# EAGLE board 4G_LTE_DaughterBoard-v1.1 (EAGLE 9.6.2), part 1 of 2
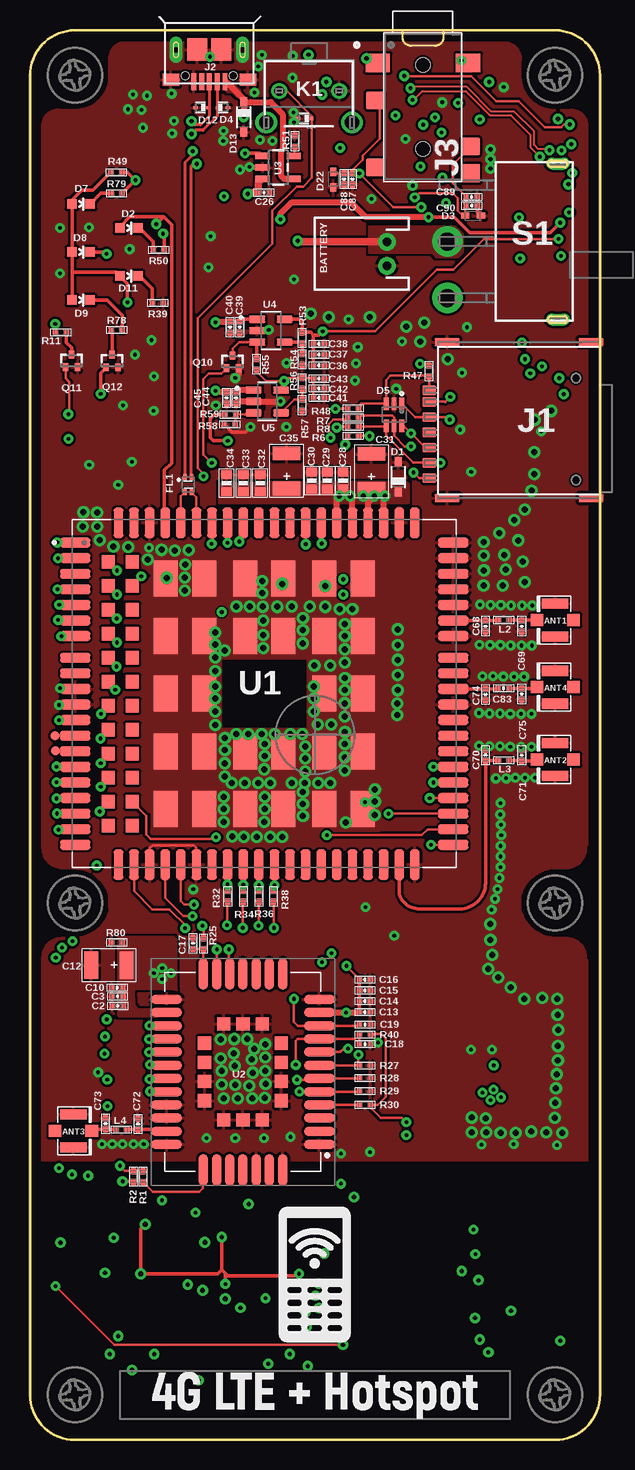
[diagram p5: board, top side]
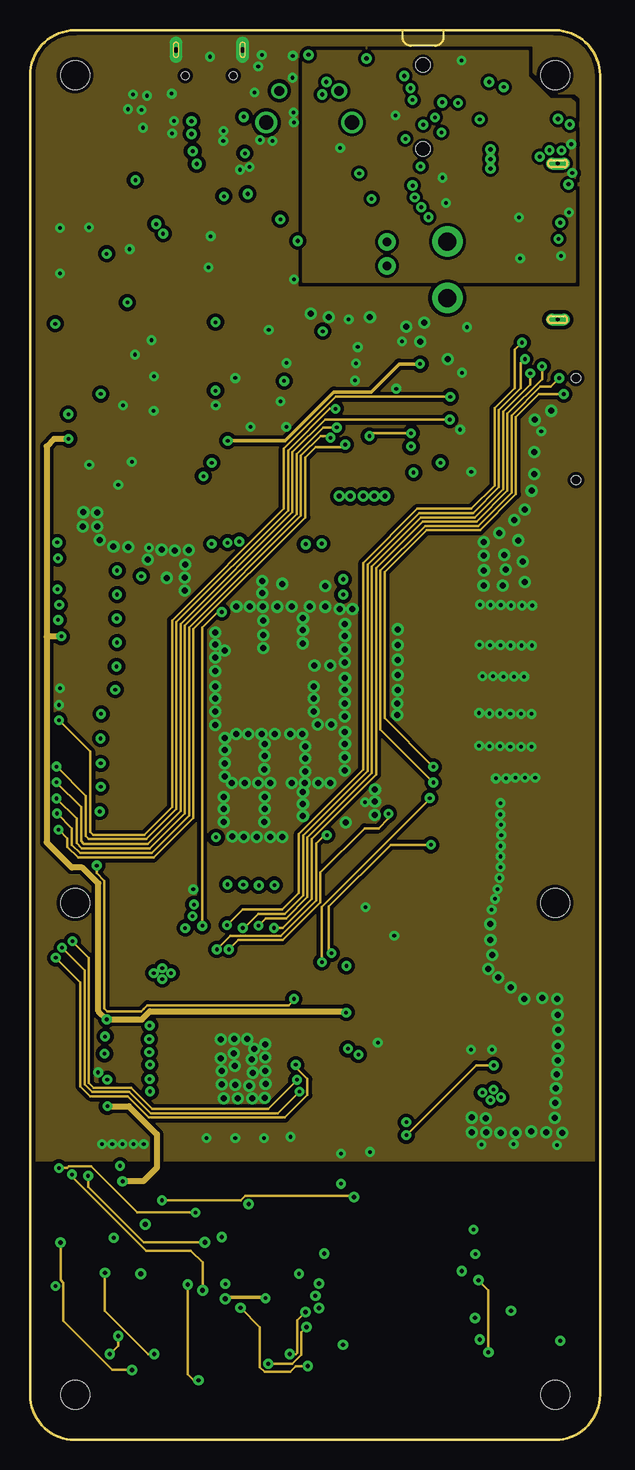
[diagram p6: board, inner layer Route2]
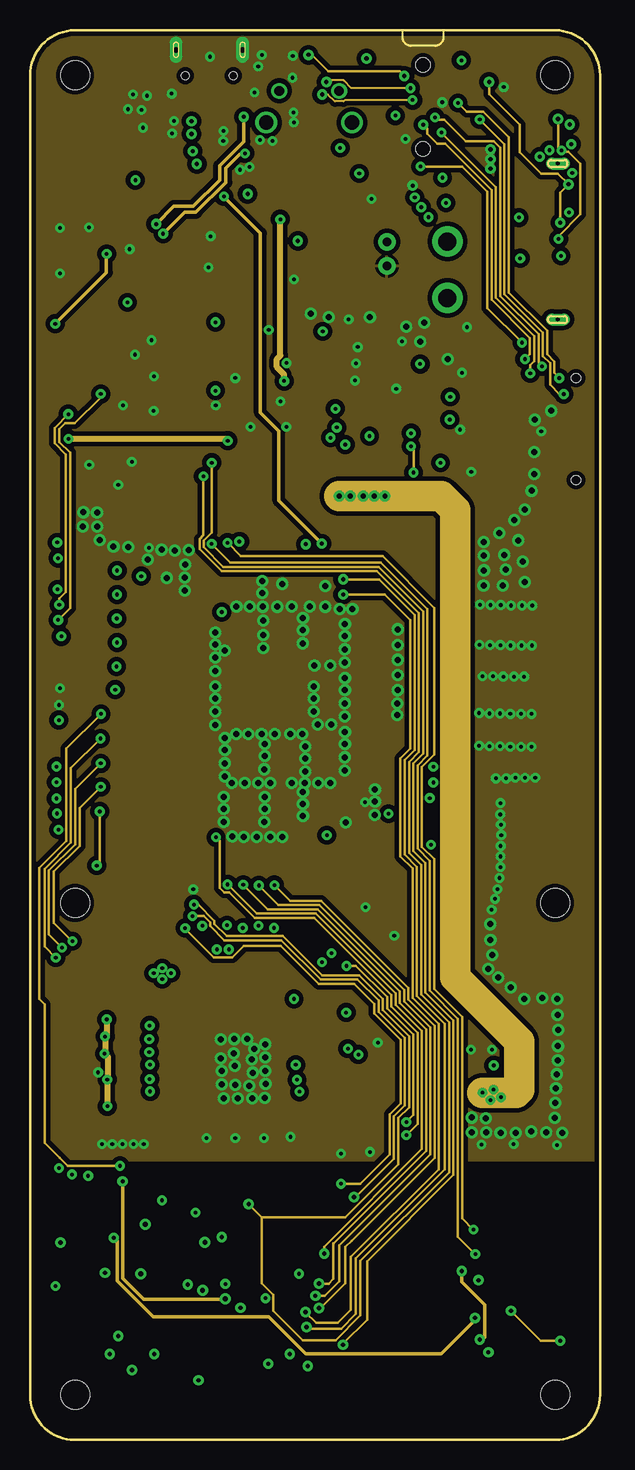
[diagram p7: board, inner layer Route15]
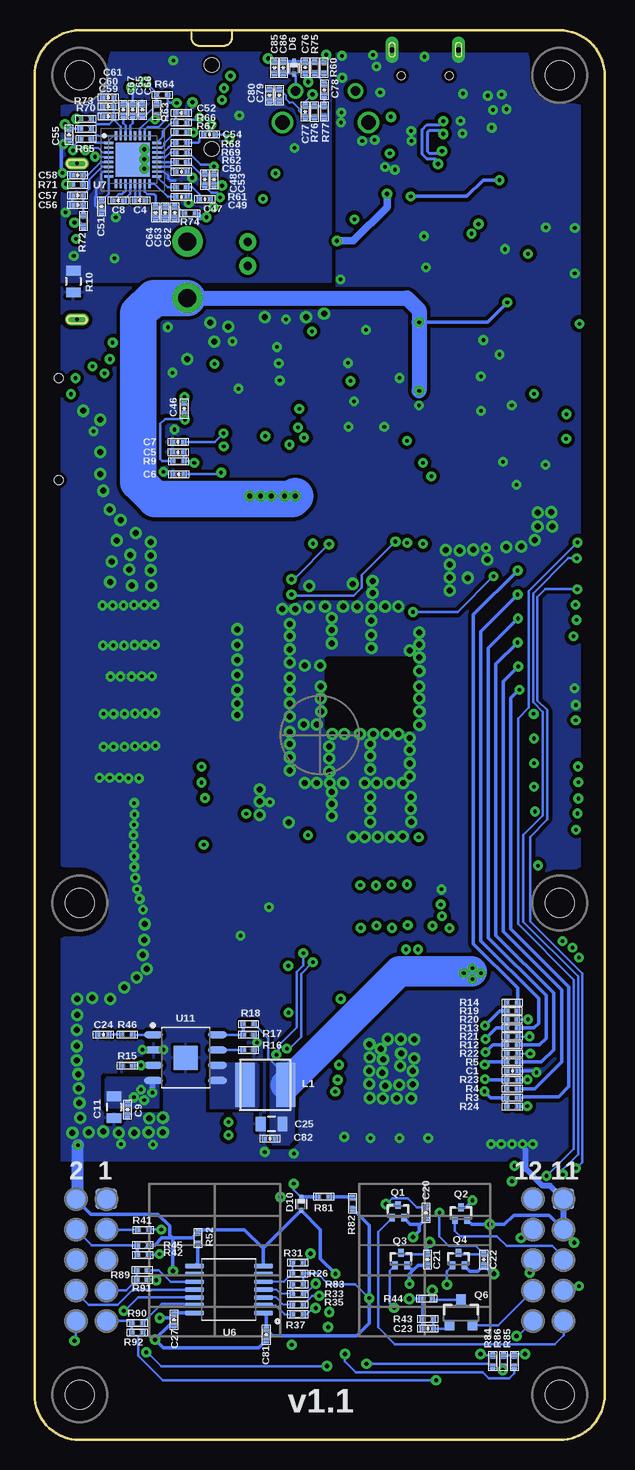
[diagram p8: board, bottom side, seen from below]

Size 47.5 x 117.5 mm. Coordinates in mm from the lower left corner, seen from the top.
Copper layers (1*2+15*16): Top 0.035mm / dielectric 1.5mm / Route2 0.035mm / dielectric 0.15mm / Route15 0.035mm / dielectric 0.2mm / Bottom 0.035mm
Design rules "4LDaughterBoards": minimum track width 6mil, minimum drill 0.3mm, track to track 6mil, track to pad 6mil, pad to pad 6mil, via to via 6mil, smd to smd 0mil, copper to edge 0.2mm, drill to drill 8mil, minimum pad ring 10mil, minimum via ring 10mil, stop-mask expansion 4mil, vias tented up to drill 25mil, thermal gap 10mil
Net classes: 1 USB_Data: width 0.261 mm, drill 0.305 mm, clearance 0.203 mm; 2 SDIO3.0: width 0.235 mm, drill 0.305 mm, clearance 0.305 mm
tRestrict: area 39.3,56.4 to 39.7,56.9; area 17.8,86.9 to 19.4,87.1; area 17.8,86 to 19.4,86.2
Milling: 5 lines

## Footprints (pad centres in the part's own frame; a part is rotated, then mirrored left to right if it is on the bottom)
U.FL = smd 2.2 x 0.85: 1 0,1.375; 2 0,-1.375 | smd 1.05 x 1: FEED 1.525,0; NC -1.525,0
JST-2-PTH = drill 0.7 pad 1.448: 1 -1,0; 2 1,0
0402-CAP = smd 0.508 x 0.508: 1 -0.457,0; 2 0.457,0
0805_CAP = smd 0.8 x 1.2: 1 -0.9,0; 2 0.9,0
AVX-B = smd 1.143 x 2.286: + -1.46,0; - 1.46,0
0603-CAP-L = smd 0.75 x 0.9: 1 -0.7,0; 2 0.7,0
SOD323 = smd 0.8 x 0.6: A 1.25,0; C -1.25,0
0603-LED = smd 0.8 x 0.8: A 0,-0.75; C 0,0.75
SOD523 = smd 0.7 x 0.5: A 0.7,0; C -0.6,0
SOD923 = smd 0.36 x 0.25: A 0.42,0; C -0.42,0
DIO_ESDA6V1-5W6 = smd 1.05 x 0.4: 1 -0.925,0.65; 2 -0.925,0; 3 -0.925,-0.65; 4 0.925,-0.65; 5 0.925,0; 6 0.925,0.65
SODFL1060X40N = smd 0.41 x 0.31: 1 -0.55,0; 2 0.55,0
SMD,1.25X1.0X0.5MM = smd 0.3 x 0.5: 1 -0.275,0.625; 2 0.275,0.625; 3 0.275,-0.625; 4 -0.275,-0.625
XUNPU-SMN-303_C266888 = smd 0.8 x 1.14: C1 0.256,7.48; C2 -2.285,7.48; C3 -4.825,7.48; C5 1.526,7.48; C6 -1.015,7.48; C7 -3.555,7.48; CD 2.476,7.48 | smd 0.7 x 2.1: P$1 -6.495,6; P$2 6.505,6; P$3 6.505,-6; P$4 -6.495,-6 | hole 0.75: -4.995,-4.75; 3.505,-4.75
B-SMD-5P-0.65SLOT = smd 0.406 x 1.4: 1 1.3,0; 2 0.65,0; 3 0,0; 4 -0.65,0; 5 -1.3,0 | smd 1.372 x 1.016: 6 -3.2,0.15; 7 3.2,0.15 | drill 0.45 pad 1.1 long: 8 2.775,2.65; 9 -2.775,2.65 | smd 1.651 x 1.9: 10 -1,2.667; 11 1,2.667 | hole 0.65: -2,0.5; 2,0.5
PJ-342-SMT_3.5MM = smd 1.524 x 2.032: 1 -3.678,-3.768; 2 -3.678,3.759 | smd 1.524 x 1.524: 3 -0.538,-3.988; 4 3.301,3.988; 5 5.037,-3.988; 6 5.52,3.988 | hole 1.2: -3.5,0; 3.51,0
3X6X5-90_DEGREE = drill 0.8: 1 -2.534,-0.964; 2 2.46,-0.964 | drill 1.2: ANCHOR1 -3.609,1.68; ANCHOR2 3.541,1.68
IND4018 = smd 1.6 x 3.7: 1 -1.7,0; 2 1.7,0
0402-IND = smd 0.508 x 0.508: 1 -0.457,0; 2 0.457,0
SC89 = smd 0.45 x 0.65: 1 -0.5,-0.525; 2 0.5,-0.525; 3 0,0.525
SOT23-3-L = smd 0.8 x 0.9: 1 -0.95,-1; 2 0.95,-1; 3 0,1.1
0402-RES = smd 0.508 x 0.508: 1 -0.457,0; 2 0.457,0
0805_RES = smd 0.8 x 1.2: 1 -0.9,0; 2 0.9,0
SWITCH_SPDT_PTH_90D_13X9.2MM = drill 1.5 pad 2.54: 2 -7.25,0; 3 -7.25,-4.7 | drill 0.3 pad 1 long: P$1 1.95,-6.5; P$2 1.95,6.5
PAD.03X.03 = smd 0.762 x 0.762: P$1 0,0
EC25EFA = smd 2.5 x 0.8: 1 -15.75,12.6; 2 -15.75,11.3; 3 -15.75,10; 4 -15.75,8.7; 5 -15.75,7.4; 6 -15.75,6.1; 7 -15.75,4.8; 8 -15.75,0.4; 9 -15.75,-0.9; 10 -15.75,-2.2; 11 -15.75,-3.5; 12 -15.75,-4.8; 13 -15.75,-6.1; 14 -15.75,-7.4; 15 -15.75,-8.7; 16 -15.75,-10; 17 -15.75,-11.3; 18 -15.75,-12.6; 37 15.75,-12.6; 38 15.75,-11.3; 39 15.75,-10; 40 15.75,-8.7; 41 15.75,-7.4; 42 15.75,-6.1; 43 15.75,-4.8; 44 15.75,-3.5; 45 15.75,-2.2; 46 15.75,-0.9; 47 15.75,0.4; 48 15.75,4.8; 49 15.75,6.1; 50 15.75,7.4; 51 15.75,8.7; 52 15.75,10; 53 15.75,11.3; 54 15.75,12.6; 141 -15.75,3; 142 -15.75,1.7; 143 15.75,1.7; 144 15.75,3 | smd 0.8 x 2.5: 19 -9.55,-14.25; 20 -8.25,-14.25; 21 -6.95,-14.25; 22 -5.65,-14.25; 23 -4.35,-14.25; 24 -3.05,-14.25; 25 -1.75,-14.25; 26 -0.45,-14.25; 27 0.85,-14.25; 28 2.15,-14.25; 29 3.45,-14.25; 30 4.75,-14.25; 31 6.05,-14.25; 32 7.35,-14.25; 33 8.65,-14.25; 34 9.95,-14.25; 35 11.25,-14.25; 36 12.55,-14.25; 55 12.55,14.25; 56 11.25,14.25; 57 9.95,14.25; 58 8.65,14.25; 59 7.35,14.25; 60 6.05,14.25; 61 4.75,14.25; 62 3.45,14.25; 63 2.15,14.25; 64 0.85,14.25; 65 -0.45,14.25; 66 -1.75,14.25; 67 -3.05,14.25; 68 -4.35,14.25; 69 -5.65,14.25; 70 -6.95,14.25; 71 -8.25,14.25; 72 -9.55,14.25; 113 -10.85,14.25; 114 -12.15,14.25; 115 -10.85,-14.25; 116 -12.15,-14.25 | smd 2 x 3: 85 8.2,9.6; 86 8.2,4.8; 87 8.2,0; 88 8.2,-4.8; 89 8.2,-9.6; 90 5,9.6; 91 5,4.8; 92 5,0; 93 5,-4.8; 94 5,-9.6; 95 1.6,9.6; 96 1.6,4.8; 97 1.6,-4.8; 98 1.6,-9.6; 99 -1.6,9.6; 100 -1.6,4.8; 101 -1.6,-4.8; 102 -1.6,-9.6; 103 -5,9.6; 104 -5,4.8; 105 -5,0; 106 -5,-4.8; 107 -5,-9.6; 108 -8.2,9.6; 109 -8.2,4.8; 110 -8.2,0; 111 -8.2,-4.8; 112 -8.2,-9.6 | smd 1.1 x 1.1: 117 -11,11; 118 -11,9; 119 -11,7; 120 -11,5; 121 -11,3; 122 -11,1; 123 -11,-1; 124 -11,-3; 125 -11,-5; 126 -11,-7; 127 -11,-9; 128 -11,-11; 129 -13,11; 130 -13,9; 131 -13,7; 132 -13,5; 133 -13,3; 134 -13,1; 135 -13,-1; 136 -13,-3; 137 -13,-5; 138 -13,-7; 139 -13,-9; 140 -13,-11
FC20N = smd 2.6 x 0.8: 1 -6.366,6.05; 2 -6.366,4.95; 3 -6.366,3.85; 4 -6.366,2.75; 5 -6.366,1.65; 6 -6.366,0.55; 7 -6.366,-0.55; 8 -6.366,-1.65; 9 -6.366,-2.75; 10 -6.366,-3.85; 11 -6.366,-4.95; 12 -6.366,-6.05; 20 6.366,-6.05; 21 6.366,-4.95; 22 6.366,-3.85; 23 6.366,-2.75; 24 6.366,-1.65; 25 6.366,-0.55; 26 6.366,0.55; 27 6.366,1.65; 28 6.366,2.75; 29 6.366,3.85; 30 6.366,4.95; 31 6.366,6.05 | smd 0.8 x 2.6: 13 -3.3,-8.166; 14 -2.2,-8.166; 15 -1.1,-8.166; 16 0,-8.166; 17 1.1,-8.166; 18 2.2,-8.166; 19 3.3,-8.166; 32 3.3,8.166; 33 2.2,8.166; 34 1.1,8.166; 35 0,8.166; 36 -1.1,8.166; 37 -2.2,8.166; 38 -3.3,8.166 | smd 1.1 x 1.1: 39 -3.2,2.4; 40 -3.2,0.8; 41 -3.2,-0.8; 42 -3.2,-2.4; 43 -1.6,-4; 44 0,-4; 45 1.6,-4; 46 3.2,-2.4; 47 3.2,-0.8; 48 3.2,0.8; 49 3.2,2.4; 50 1.6,4; 51 0,4; 52 -1.6,4
SOT23-5 = smd 0.55 x 1.2: 1 -0.95,-1.3; 2 0,-1.3; 3 0.95,-1.3; 4 0.95,1.3; 5 -0.95,1.3
SOT23-5(SOT95P280X145-5N) = smd 1.32 x 0.59: 1 -1.145,0.95; 2 -1.145,0; 3 -1.145,-0.95; 4 1.145,-0.95; 5 1.145,0.95
SOP65P640X120-14N = smd 1.57 x 0.41: 1 -2.87,1.95; 2 -2.87,1.3; 3 -2.87,0.65; 4 -2.87,0; 5 -2.87,-0.65; 6 -2.87,-1.3; 7 -2.87,-1.95; 8 2.87,-1.95; 9 2.87,-1.3; 10 2.87,-0.65; 11 2.87,0; 12 2.87,0.65; 13 2.87,1.3; 14 2.87,1.95
QFN40P400X400X90-33N = smd 0.75 x 0.2: 1 -2,1.4; 2 -2,1; 3 -2,0.6; 4 -2,0.2; 5 -2,-0.2; 6 -2,-0.6; 7 -2,-1; 8 -2,-1.4; 17 2,-1.4; 18 2,-1; 19 2,-0.6; 20 2,-0.2; 21 2,0.2; 22 2,0.6; 23 2,1; 24 2,1.4 | smd 0.2 x 0.75: 9 -1.4,-2; 10 -1,-2; 11 -0.6,-2; 12 -0.2,-2; 13 0.2,-2; 14 0.6,-2; 15 1,-2; 16 1.4,-2; 25 1.4,2; 26 1,2; 27 0.6,2; 28 0.2,2; 29 -0.2,2; 30 -0.6,2; 31 -1,2; 32 -1.4,2 | smd 2.85 x 2.85: 33 0,0
SOP-8-150MIL(SOIC127P600X175-8T200) = smd 1.585 x 0.602: 1 -2.665,1.905; 2 -2.665,0.635; 3 -2.665,-0.635; 4 -2.665,-1.905; 5 2.665,-1.905; 6 2.665,-0.635; 7 2.665,0.635; 8 2.665,1.905 | smd 2 x 2: 9 0,0
WIPHONE_DAUGHTERBOARD = smd 1.75 x 1.75 bottom: 1 17.78,-38.66; 2 20.32,-38.66; 3 17.78,-41.2; 4 20.32,-41.2; 5 17.78,-43.74; 6 20.32,-43.74; 7 17.78,-46.28; 8 20.32,-46.28; 9 17.78,-48.82; 10 20.32,-48.82; 11 -20.32,-38.66; 12 -17.78,-38.66; 13 -20.32,-41.2; 14 -17.78,-41.2; 15 -20.32,-43.74; 16 -17.78,-43.74; 17 -20.32,-46.28; 18 -17.78,-46.28; 19 -20.32,-48.82; 20 -17.78,-48.82 | hole 2.4: 20,-54.991; -20,-54.991; 20,-13.991; 20,55.009; -20,55.009; -20,-13.991

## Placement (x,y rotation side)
ANT1  IPEX connector  [U.FL]  43.76,68.34 180 top
ANT2  IPEX connector  [U.FL]  43.76,56.7 180 top
ANT3  IPEX connector  [U.FL]  3.62,25.75 0 top
ANT4  IPEX connector  [U.FL]  43.76,62.74 180 top
BATTERY  MOLEX_BATT_2JST-PTH-2  [JST-2-PTH]  29.75,98.86 90 top
C1  NC  [0402-CAP]  7.69,30.75 0 bottom
C2  10pF  [0402-CAP]  7.31,36.17 0 top
C3  33pF  [0402-CAP]  7.29,36.96 0 top
C4  2.2uF  [0402-CAP]  38.73,103.32 180 bottom
C5  33pF  [0402-CAP]  35.54,82.33 180 bottom
C6  33pF  [0402-CAP]  35.49,80.49 180 bottom
C7  33pF  [0402-CAP]  35.54,83.18 180 bottom
C8  2.2uF  [0402-CAP]  40.53,103.32 180 bottom
C9  0.1uF  [0402-CAP]  39.76,27.53 90 bottom
C10  100nF  [0402-CAP]  7.27,37.69 0 top
C11  22uF  [0805_CAP]  40.89,27.73 270 bottom
C12  100uF  [AVX-B]  6.57,39.58 180 top
C13  10pF  [0402-CAP]  27.91,35.66 180 top
C14  33pF  [0402-CAP]  27.91,36.56 180 top
C15  100nF  [0402-CAP]  27.91,37.46 180 top
C16  10uF  [0402-CAP]  27.91,38.36 180 top
C17  NC  [0402-CAP]  13.58,41.38 270 top
C18  100nF  [0402-CAP]  27.91,32.99 0 top
C19  NC  [0402-CAP]  27.91,34.62 0 top
C20  10nF  [0402-CAP]  14.88,18.92 270 bottom
C21  10nF  [0402-CAP]  14.78,15.02 270 bottom
C22  10nF  [0402-CAP]  10.08,15.02 270 bottom
C23  1nF  [0402-CAP]  14.74,9.26 0 bottom
C24  560pF  [0402-CAP]  41.78,33.79 0 bottom
C25  22uF  [0805_CAP]  27.76,26.32 180 bottom
C26  4.7uF  [0402-CAP]  19.48,103.96 0 top
C27  10nF  [0402-CAP]  35.9,10 270 bottom
C28  10pF  [0603-CAP-L]  26.08,79.96 270 top
C29  33pF  [0603-CAP-L]  24.78,79.96 270 top
C30  100nF  [0603-CAP-L]  23.48,79.96 270 top
C31  100uF  [AVX-B]  28.45,80.72 90 top
C32  10pF  [0603-CAP-L]  19.18,79.76 270 top
C33  33pF  [0603-CAP-L]  17.78,79.76 270 top
C34  100nF  [0603-CAP-L]  16.38,79.76 270 top
C35  100uF  [AVX-B]  21.38,80.76 90 top
C36  33pF  [0402-CAP]  24.08,89.56 180 top
C37  100nF  [0402-CAP]  24.08,90.46 180 top
C38  4.7uF  [0402-CAP]  24.08,91.36 180 top
C39  100nF  [0402-CAP]  17.48,92.76 90 top
C40  1uF  [0402-CAP]  16.68,92.76 90 top
C41  33pF  [0402-CAP]  24.08,86.86 180 top
C42  100nF  [0402-CAP]  24.08,87.66 180 top
C43  4.7uF  [0402-CAP]  24.08,88.46 180 top
C44  100nF  [0402-CAP]  17.18,86.86 90 top
C45  1uF  [0402-CAP]  16.38,86.86 90 top
C46  100nF  [0402-CAP]  35.04,85.97 90 bottom
C47  1uF  [0402-CAP]  33.33,103.42 0 bottom
C48  1uF  [0402-CAP]  33.33,105.06 270 bottom
C49  2.2uF  [0402-CAP]  35.28,103.62 0 bottom
C50  2.2uF  [0402-CAP]  35.28,105.72 0 bottom
C51  4.7uF  [0402-CAP]  41.93,102.82 270 bottom
C52  NC  [0402-CAP]  35.28,110.61 180 bottom
C53  NC  [0402-CAP]  32.55,105.07 90 bottom
C54  NC  [0402-CAP]  32.93,108.82 180 bottom
C55  4.7uF  [0402-CAP]  44.65,108.79 270 bottom
C56  100nF  [0402-CAP]  43.93,102.93 0 bottom
C57  4.7uF  [0402-CAP]  43.93,103.72 0 bottom
C58  4.7uF  [0402-CAP]  43.93,105.42 0 bottom
C59  100nF  [0402-CAP]  41.38,110.31 0 bottom
C60  4.7uF  [0402-CAP]  41.38,111.14 0 bottom
C61  NC  [0402-CAP]  41.38,111.89 0 bottom
C62  33pF  [0402-CAP]  35.83,102.32 90 bottom
C63  100nF  [0402-CAP]  36.63,102.32 90 bottom
C64  4.7uF  [0402-CAP]  37.43,102.32 90 bottom
C65  100nF  [0402-CAP]  39.33,110.86 270 bottom
C66  2.2uF  [0402-CAP]  38.53,110.86 270 bottom
C67  2.2uF  [0402-CAP]  40.13,110.86 270 bottom
C68  NC  [0402-CAP]  37.97,67.84 90 top
C69  NC  [0402-CAP]  40.98,67.84 90 top
C70  NC  [0402-CAP]  37.97,57.07 270 top
C71  NC  [0402-CAP]  40.98,57.06 270 top
C72  NC  [0402-CAP]  9,26.32 270 top
C73  NC  [0402-CAP]  6.29,26.35 270 top
C74  NC  [0402-CAP]  37.97,62.14 90 top
C75  NC  [0402-CAP]  40.98,62.18 90 top
C76  2.2uF  [0402-CAP]  24.95,114.38 270 bottom
C77  2.2uF  [0402-CAP]  24.95,110.73 90 bottom
C78  2.2uF  [0402-CAP]  23.37,112.53 90 bottom
C79  4.7uF  [0402-CAP]  27.12,112.09 90 bottom
C80  33pF  [0402-CAP]  27.93,112.09 90 bottom
C81  10nF  [0402-CAP]  28.2,8.76 270 bottom
C82  0.1uF  [0402-CAP]  27.9,25.1 0 bottom
C83  100pF  [0402-CAP]  39.47,62.64 180 top
C85  10pF  [0402-CAP]  27.52,114.38 90 bottom
C86  33pF  [0402-CAP]  26.78,114.38 90 bottom
C87  10pF  [0402-CAP]  26.88,105.1 90 top
C88  33pF  [0402-CAP]  26.18,105.1 90 top
C89  10pF  [0402-CAP]  36.81,103.62 180 top
C90  33pF  [0402-CAP]  36.82,102.88 180 top
D1  PZ3D4V2H  [SOD323]  30.68,80.26 90 top
D2  RED  [0603-LED]  8.25,101.02 270 top
D3  LESD5D5.0CT1G  [SOD523]  36.87,102.03 0 top
D4  ESD9L5.0ST5G  [SOD923]  16.08,111.06 0 top
D5  ESDA6V1-5W6  [DIO_ESDA6V1-5W6]  30.34,85.44 270 top
D6  ESD9X5.0ST5G  [SODFL1060X40N]  25.9,114.37 270 bottom
D7  Green  [0603-LED]  4.25,103.02 270 top
D8  RED  [0603-LED]  4.25,99.02 270 top
D9  Green  [0603-LED]  4.25,95.02 270 top
D10  ESD9X3.3ST5G  [SODFL1060X40N]  25.29,19.66 270 bottom
D11  Green  [0603-LED]  8.25,97.02 270 top
D12  ESD9L5.0ST5G  [SOD923]  14.22,111.06 180 top
D13  SD12  [SOD323]  17.82,110.26 270 top
D14  ESD9X3.3ST5G  [SODFL1060X40N]  22.85,110.14 180 top
D22  LESD5D5.0CT1G  [SOD523]  25.28,105.1 270 top
FL1  [SMD,1.25X1.0X0.5MM]  13.18,79.63 0 top
J1  XUNPU-SMN-3031  [XUNPU-SMN-303_C266888]  40.75,85 90 top
J2  MICRO_USB_5P_TH-JLC  [B-SMD-5P-0.65SLOT]  14.95,113.22 0 top
J3  PJ-342-SMT_3.5MM  [PJ-342-SMT_3.5MM]  32.75,111.11 270 top
K1  [3X6X5-90_DEGREE]  23.23,111.49 180 top
L1  3.3uH/2A  [IND4018]  28.28,29.59 0 bottom
L2  0R  [0402-IND]  39.47,68.34 0 top
L3  0R  [0402-IND]  39.47,56.64 0 top
L4  0R  [0402-IND]  7.62,25.85 180 top
Q1  DTC043ZEBTL  [SC89]  17.22,19.04 0 bottom
Q2  DTC043ZEBTL  [SC89]  11.98,18.86 0 bottom
Q3  DTC043ZEBTL  [SC89]  16.98,15.06 0 bottom
Q4  DTC043ZEBTL  [SC89]  12.18,15.06 0 bottom
Q6  2SC4617TLQ  [SOT23-3-L]  11.98,10.56 0 bottom
Q10  DTC043ZEBTL  [SC89]  16.88,89.86 0 top
Q11  DTC043ZEBTL  [SC89]  3.46,89.94 0 top
Q12  DTC043ZEBTL  [SC89]  6.85,89.93 0 top
R1  0R  [0402-RES]  9.42,21.95 270 top
R2  10k  [0402-RES]  8.62,21.95 90 top
R3  0R  [0402-RES]  7.7,28.52 180 bottom
R4  0R  [0402-RES]  7.7,29.26 180 bottom
R5  0R  [0402-RES]  7.7,31.48 180 bottom
R6  0R  [0402-RES]  26.94,83.69 180 top
R7  0R  [0402-RES]  26.94,85.21 180 top
R8  0R  [0402-RES]  26.94,84.46 180 top
R9  15k  [0402-RES]  35.52,81.58 0 bottom
R10  0R  [0805_RES]  44.28,96.56 270 bottom
R11  2.2k  [0402-RES]  2.57,92.33 0 top
R12  0R  [0402-RES]  7.72,32.91 180 bottom
R13  0R  [0402-RES]  7.71,34.32 180 bottom
R14  0R  [0402-RES]  7.71,36.45 180 bottom
R15  100k  [0402-RES]  39.78,31.19 180 bottom
R16  330k  [0402-RES]  29.68,32.49 0 bottom
R17  24k 1%  [0402-RES]  29.68,33.76 0 bottom
R18  75k 1%  [0402-RES]  29.68,34.66 180 bottom
R19  NC  [0402-RES]  7.72,35.75 0 bottom
R20  10k  [0402-RES]  7.72,35.04 0 bottom
R21  NC  [0402-RES]  7.7,33.62 0 bottom
R22  NC  [0402-RES]  7.71,32.2 0 bottom
R23  NC  [0402-RES]  7.69,30.02 0 bottom
R24  NC  [0402-RES]  7.69,27.78 0 bottom
R25  0R  [0402-RES]  14.46,41.36 270 top
R26  10k  [0402-RES]  25.58,13.86 0 bottom
R27  10k  [0402-RES]  27.91,31.19 0 top
R28  10k  [0402-RES]  27.91,30.15 0 top
R29  15k  [0402-RES]  27.91,29.07 0 top
R30  10k  [0402-RES]  27.91,27.92 0 top
R31  NC  [0402-RES]  25.58,14.76 0 bottom
R32  0R  [0402-RES]  16.48,45.3 90 top
R33  NC  [0402-RES]  25.58,12.16 0 bottom
R34  0R  [0402-RES]  17.78,45.3 90 top
R35  NC  [0402-RES]  25.58,11.26 0 bottom
R36  0R  [0402-RES]  19.08,45.3 90 top
R37  NC  [0402-RES]  25.58,10.46 0 bottom
R38  0R  [0402-RES]  20.28,45.3 90 top
R39  2.2k  [0402-RES]  10.65,94.77 0 top
R40  NC  [0402-RES]  27.91,33.76 0 top
R41  1k  [0402-RES]  38.46,17.49 0 bottom
R42  1k  [0402-RES]  38.49,15.41 0 bottom
R43  4.7k  [0402-RES]  14.74,10.06 0 bottom
R44  4.7k  [0402-RES]  14.84,11.76 0 bottom
R45  15k  [0402-RES]  38.49,16.23 0 bottom
R46  39k  [0402-RES]  39.78,33.79 180 bottom
R47  51k  [0402-RES]  33.24,89.09 270 top
R48  0R  [0402-RES]  26.94,85.97 180 top
R49  10K  [0402-RES]  7.2,105.66 0 top
R50  1k  [0402-RES]  10.73,99.19 180 top
R51  2k  [0402-RES]  22.08,108.26 270 top
R52  4.7K  [0402-RES]  33.9,16.82 270 bottom
R53  73.2k 1%  [0402-RES]  22.68,91.86 270 top
R54  42.2k 1%  [0402-RES]  22.68,90.06 270 top
R55  10k  [0402-RES]  18.88,89.66 270 top
R56  39k 1%  [0402-RES]  22.68,88.06 270 top
R57  75k 1%  [0402-RES]  22.68,86.26 270 top
R58  100k  [0402-RES]  16.65,84.66 180 top
R59  0R  [0402-RES]  16.68,85.46 0 top
R60  1k  [0402-RES]  23.39,114.38 270 bottom
R61  0R  [0402-RES]  35.28,104.42 180 bottom
R62  0R  [0402-RES]  35.28,106.52 180 bottom
R63  4.7k  [0402-RES]  37.33,110.86 90 bottom
R64  4.7k  [0402-RES]  36.88,112.11 180 bottom
R65  NC  [0402-RES]  43.23,108.43 180 bottom
R66  0R  [0402-RES]  35.28,109.81 0 bottom
R67  0R  [0402-RES]  35.28,109.02 0 bottom
R68  0R  [0402-RES]  35.28,108.12 0 bottom
R69  0R  [0402-RES]  35.28,107.32 0 bottom
R70  0R  [0402-RES]  43.24,109.28 0 bottom
R71  0R  [0402-RES]  43.93,104.62 0 bottom
R72  0R  [0402-RES]  43.43,101.61 90 bottom
R73  0R  [0402-RES]  43.24,110.11 0 bottom
R74  0R  [0402-RES]  34.55,102.24 180 bottom
R75  1.5k  [0402-RES]  24.16,114.38 90 bottom
R76  1.5k  [0402-RES]  24.19,110.72 90 bottom
R77  1k  [0402-RES]  23.37,110.73 270 bottom
R78  2.2k  [0402-RES]  7.23,92.52 180 top
R79  2.2k  [0402-RES]  7.21,103.91 0 top
R80  51k  [0402-RES]  7.23,41.46 0 top
R81  NC  [0402-RES]  23.41,20.27 180 bottom
R82  4.7k  [0402-RES]  21.01,19.71 90 bottom
R83  10k  [0402-RES]  25.58,12.96 0 bottom
R84  1k  [0402-RES]  9.33,6.57 270 bottom
R85  1k  [0402-RES]  7.53,6.57 270 bottom
R86  15k  [0402-RES]  8.43,6.57 270 bottom
R89  0R  [0402-RES]  38.55,14.14 0 bottom
R90  0R  [0402-RES]  38.95,9.74 0 bottom
R91  NC  [0402-RES]  38.55,13.34 0 bottom
R92  NC  [0402-RES]  38.95,8.94 0 bottom
S1  [SWITCH_SPDT_PTH_90D_13X9.2MM]  42.03,99.89 0 top
TP1  TEST-POINT3  [PAD.03X.03]  2.09,58.69 0 top
TP2  TEST-POINT3  [PAD.03X.03]  2.12,57.43 0 top
U1  EC25  [EC25EFA]  19.52,62.2 0 top
U2  FC20  [FC20N]  17.75,30.67 180 top
U3  MCP73831  [SOT23-5]  20.68,106.06 270 top
U4  SGM2019-ADJYN5G/TR  [SOT23-5(SOT95P280X145-5N)]  20.08,92.46 0 top
U5  SGM2019-ADJYN5G/TR  [SOT23-5(SOT95P280X145-5N)]  19.78,86.56 0 top
U6  TXS0104EPWR  [SOP65P640X120-14N]  31.32,12.52 180 bottom
U7  ALC5616  [QFN40P400X400X90-33N]  39.33,106.72 0 bottom
U11  RT8074  [SOP-8-150MIL(SOIC127P600X175-8T200)]  34.93,31.85 0 bottom
WIPHONE_DAUGHTERBOARD-FOOTPRINT1  WIPHONE_DAUGHTERBOARD  [WIPHONE_DAUGHTERBOARD]  23.75,58.74 0 top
